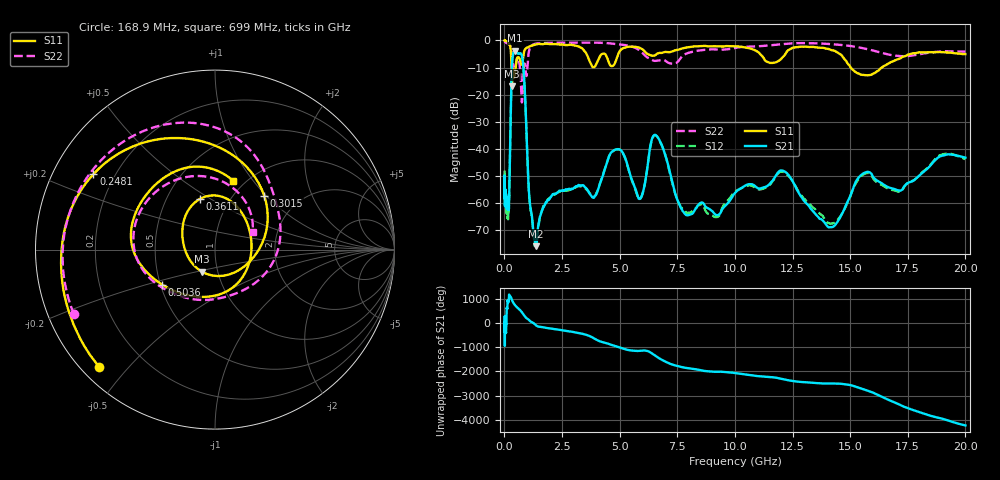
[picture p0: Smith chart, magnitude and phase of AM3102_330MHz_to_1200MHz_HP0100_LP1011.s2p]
! Date/Time: Tue, Sep 11, 2018 5:13 PM
! Network Analyzer: Agilent Technologies E8362B Rev: A.07.50.63
! Sweep from 0.010 to 20.000 GHz, 1601 Points, Sweep Type: LOG
! Power Supply: 4.949 V, 0.001 A
# Hz S DB R 50
!freq MagS11 AngS11 MagS21 AngS21 MagS12 AngS12 MagS22 AngS22
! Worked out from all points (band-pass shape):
!   1601 points, 10 MHz to 20 GHz, reference 50 ohm
!   highest |S21| = -3.75 dB at 464.5 MHz (marker M1); lowest = -75.9 dB at 1.353 GHz (marker M2)
!   |S21| within 3 dB of the highest: 347.5 MHz to 786.5 MHz (439 MHz wide, 77.4 % of centre)
!   lowest |S11| = -16.9 dB at 330 MHz (marker M3), VSWR 1.33, Z = 42.1 - j10.6 ohm
!   |S11| at or under -10 dB: 308 MHz to 492.1 MHz (184.2 MHz wide, 46 % of centre); 15.03 GHz to 16.37 GHz (1.347 GHz wide, 8.58 % of centre)
!   |S22| runs from -22.9 to -0.3 dB; largest |S21 - S12| = 0.012
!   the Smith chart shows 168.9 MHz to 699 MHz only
!   S11 on the Smith chart (normalised r, x): 168.9 MHz: 0.05, -0.42; 248.1 MHz: 0.12, +0.28; 301.5 MHz: 1.35, +0.97; 361.1 MHz: 0.73, +0.45; 503.6 MHz: 0.51, -0.23; 699 MHz: 0.89, +0.80
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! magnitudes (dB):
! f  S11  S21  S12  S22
! 10 MHz  0.0  -50.0  -48.0  -0.3
! 35.55 MHz  0.0  -58.1  -59.1  -0.5
! 126.4 MHz  -0.4  -59.8  -62.9  -1.1
! 168.9 MHz  -0.7  -62.3  -64.5  -1.3
! 248.1 MHz  -2.0  -40.1  -40.1  -1.9
! 301.5 MHz  -7.8  -16.4  -16.4  -3.6
! 330 MHz  -16.9  -8.8  -8.8  -6.2
! 361.1 MHz  -10.6  -5.9  -6.0  -8.5
! 447.2 MHz  -12.8  -3.8  -3.8  -10.7
! 464.5 MHz  -11.9  -3.8  -3.8  -10.1
! 503.6 MHz  -9.0  -3.9  -4.1  -8.3
! 699 MHz  -8.1  -4.8  -4.8  -12.7
! 841.2 MHz  -4.8  -11.8  -11.9  -10.4
! 1.353 GHz  -1.5  -75.9  -75.2  -1.2
! 1.59 GHz  -1.4  -63.9  -63.8  -1.0
! 4.855 GHz  -7.1  -40.2  -40.3  -1.3
! 5.652 GHz  -2.3  -54.0  -54.5  -2.6
! 6.612 GHz  -5.0  -35.3  -35.3  -7.5
! 7.882 GHz  -2.6  -64.4  -63.4  -4.9
! 12.03 GHz  -6.6  -48.0  -48.4  -1.4
! 14.07 GHz  -3.2  -69.0  -67.4  -1.3
! 20 GHz  -5.0  -43.3  -43.9  -4.1
